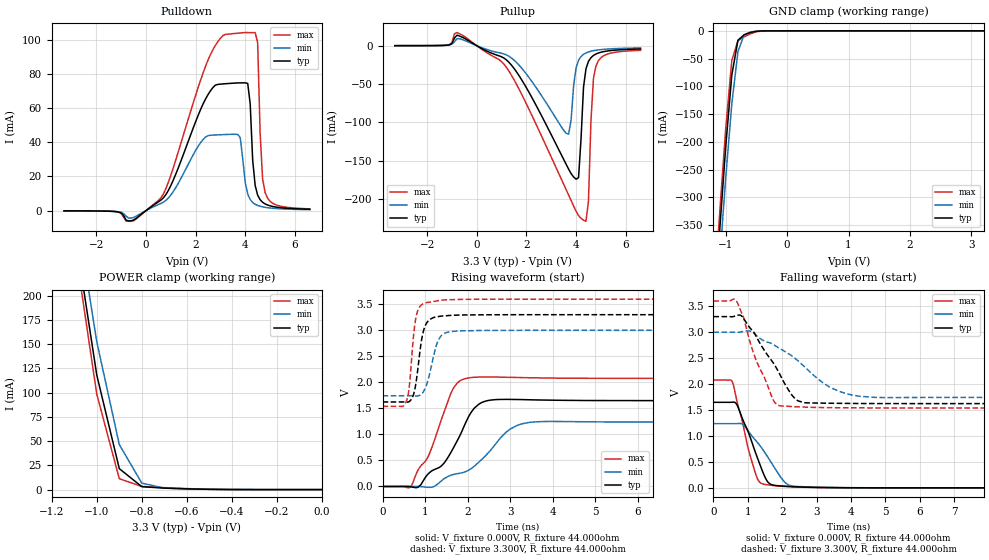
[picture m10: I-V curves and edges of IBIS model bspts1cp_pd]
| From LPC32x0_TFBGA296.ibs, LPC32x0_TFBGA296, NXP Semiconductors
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| |   Rev 0.20 IBIS Model Design Automation Generation   |
| |   N O N - S I L I C O N   C O R R E L A T E D   |
| |   This IBIS [Model] is pre-Beta tactical support   |
| |  Note: this IBIS [Model] contains clamp curves generated   |
| |   through simulation which should not be relied upon   |
| bspts1cp
|   Bidirectional Pad 3v3
|   3state Output
|   Plain Input
|   1ns Slew Rate control
|   CMOS
|   Programmable between
|   - (p1=0, p2=1) plain input
|   - (p1=0, p2=0) with Pull Up
|   - (p1=1, p2=1) with Pull Down
|   - (p1=1, p2=0) with Repeater
|   Characterized at Core 1.2V and I/O 3.3V
| Pull Down Mode (p1=1, p2=1)
[Model]   bspts1cp_pd | of bspts1cp
Model_type   I/O
Polarity   Non-Inverting
Enable   Active-Low
|  Reciever Thresholds
Vinl   = 0.36V
Vinh   = 0.84V
| AC Test Load Conditions
Vref   = 0
Cref   = 1.2e-11
Rref   = 1000000000
Vmeas   = 0.6
| [Process Range]   typical   min   max
| C_comp edge width   400.000ps   400.000ps   400.000ps
| C_comp Tstrobe   40.000fs   40.000fs   40.000fs
C_comp   2.380pF   2.240pF   2.550pF
[Temperature Range]   25   125   -40
[Voltage Range]   3.30V   3.00V   3.60V
[GND Clamp Reference]   0.00V   0.00V   0.00V
[Pulldown Reference]   0.00V   0.00V   0.00V
[POWER Clamp Reference]   3.30V   3.00V   3.60V
[Pullup Reference]   3.30V   3.00V   3.60V
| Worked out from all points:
|   slope of the pulldown table from 0 to 0.495 V, typ, clamps not added: 97.1 ohm
|   slope of the pullup table from 0 to 0.495 V, typ, clamps not added: 59.3 ohm
|   GND clamp passes 1 mA (typ) near -0.51 V on its own axis
|   POWER clamp passes 1 mA (typ) near -0.63 V on its own axis
|   rising waveform, V_fixture 0.000V, R_fixture 44.000ohm: 20-80 % time 779ps typ, 1.07ns min, 628ps max; typ from 0 V to 1.65 V
|   falling waveform, V_fixture 0.000V, R_fixture 44.000ohm: 20-80 % time 570ps typ, 781ps min, 474ps max; typ from 1.65 V to 0 V
|   rising waveform, V_fixture 3.300V, R_fixture 44.000ohm: 20-80 % time 175ps typ, 231ps min, 140ps max; typ from 1.62 V to 3.3 V
|   falling waveform, V_fixture 3.300V, R_fixture 44.000ohm: 20-80 % time 911ps typ, 1.48ns min, 670ps max; typ from 3.3 V to 1.62 V
[GND Clamp]
| ref voltage   0.00V   0.00V   0.00V
|   Voltage   I(typ)   I(min)   I(max)
-3.3V     -4.198A    -4.223A    -4.188A
-1.2V     -526mA     -577.5mA   -497.2mA
-1.1V     -363.6mA   -417.9mA   -332.6mA
-1V       -210.1mA   -266.3mA   -177.3mA
-900mV    -79.71mA   -131.5mA   -53.29mA
-800mV    -16.76mA   -37.38mA   -17.81mA
-700mV    -7.164mA   -7.263mA   -10.92mA
-600mV    -3.002mA   -2.202mA   -5.445mA
-500mV    -699uA     -571.9uA   -1.612mA
-400mV    -79uA      -96.04uA   -163.6uA
3.2V      50.82uA    25.42uA    83.99uA
[Power Clamp]   | Vtable = Vcc - Vpad
| ref voltage   3.30V   3.00V   3.60V
|   Voltage   I(typ)   I(min)   I(max)
-3.3V     4.52A      4.504A     4.537A
-1.1V     269.9mA    299.6mA    255.3mA
-1V       118.1mA    152.4mA    98.48mA
-900mV    21.62mA    46.52mA    11.25mA
-800mV    3.036mA    6.671mA    3.29mA
-700mV    1.546mA    1.556mA    2.017mA
-600mV    791.6uA    711.6uA    1.06mA
-400mV    91.28uA    94.64uA    124.4uA
0V        50.84uA    24.87uA    84.1uA
[Pulldown]
| ref voltage   0.00V   0.00V   0.00V
|   Voltage   I(typ)   I(min)   I(max)
-3.3V     -80.68uA   -69.9uA    -74.32uA
-600mV    -5.92mA    -4.329mA   -6.172mA
500mV     5.147mA    3.568mA    5.922mA
2.5V      67.8mA     43.83mA    87.99mA
3.7V      74.65mA    44.53mA    103.7mA
4V        74.69mA    16.44mA    104.1mA
4.2V      62.38mA    6.515mA    104mA
4.3V      29.48mA    4.769mA    104mA
4.5V      9.069mA    3.068mA    98.17mA
4.6V      6.413mA    2.587mA    45.15mA
4.8V      3.956mA    1.96mA     10.6mA
6.6V      844.8uA    597.5uA    1.056mA
[Pullup]   | Vtable = Vcc - Vpad
| ref voltage   3.30V   3.00V   3.60V
|   Voltage   I(typ)   I(min)   I(max)
-3.3V     39.4uA     37.84uA    38.83uA
-800mV    13.66mA    9.123mA    17.15mA
1V        -14.52mA   -9.936mA   -20.86mA
3.7V      -161.3mA   -115.5mA   -195.1mA
4V        -174.4mA   -29.02mA   -216.2mA
4.1V      -172.4mA   -19.17mA   -221.9mA
4.4V      -30.01mA   -9.422mA   -229.4mA
4.5V      -20.39mA   -8.135mA   -202.5mA
4.6V      -15.6mA    -7.195mA   -97.92mA
4.7V      -12.75mA   -6.48mA    -42.98mA
4.8V      -10.87mA   -5.92mA    -26.67mA
6.6V      -4.278mA   -2.929mA   -6.056mA
[Ramp]
R_load   = 44.000ohm
|   dV/dt(typ)   dV/dt(min)   dV/dt(max)
dV/dt_r   1.003V/795.000ps   754.478mV/1.100ns   1.260V/635.000ps
dV/dt_f   1.021V/900.000ps   769.240mV/1.445ns   1.253V/655.000ps
[Rising Waveform]  | cubic spline decimation from 2001 points
V_fixture   = 0.000V
R_fixture   = 44.000ohm
|   Time   V(typ)   V(min)   V(max)
0s        20.64nV    394.3nV    10.69nV
655ps     -4.509mV   428.1uV    -8.81mV
1.09ns    255.6mV    -17.26mV   603.8mV
1.445ns   447.6mV    146.5mV    1.426V
1.67ns    745mV      230.7mV    1.89V
1.965ns   1.242V     288.3mV    2.076V
2.37ns    1.625V     548.9mV    2.103V
2.915ns   1.673V     1.048V     2.097V
3.41ns    1.666V     1.225V     2.089V
10ns      1.648V     1.237V     2.076V
[Falling Waveform]  | cubic spline decimation from 2001 points
V_fixture   = 0.000V
R_fixture   = 44.000ohm
|   Time   V(typ)   V(min)   V(max)
0s        1.648V     1.237V     2.076V
555ps     1.65V      1.237V     2.038V
695ps     1.587V     1.238V     1.641V
1.075ns   967.6mV    1.04V      606.4mV
1.28ns    579.3mV    875mV      177mV
1.425ns   325.8mV    749.7mV    78.35mV
1.675ns   66.27mV    496.9mV    50.08mV
2.08ns    31.91mV    105.1mV    27.13mV
2.34ns    22mV       31.75mV    18.32mV
10ns      525.7nV    1.302uV    537.6nV
[Rising Waveform]  | cubic spline decimation from 2001 points
V_fixture   = 3.300V
V_fixture_min = 3.000V
V_fixture_max = 3.600V
R_fixture   = 44.000ohm
|   Time   V(typ)   V(min)   V(max)
0s        1.623V     1.742V     1.539V
555ps     1.622V     1.742V     1.629V
630ps     1.632V     1.742V     1.925V
730ps     1.769V     1.741V     2.902V
785ps     1.98V      1.739V     3.24V
920ps     2.821V     1.777V     3.49V
1.005ns   3.09V      1.889V     3.524V
1.31ns    3.263V     2.804V     3.57V
1.59ns    3.285V     2.972V     3.587V
10ns      3.299V     2.999V     3.598V
[Falling Waveform]  | cubic spline decimation from 2001 points
V_fixture   = 3.300V
V_fixture_min = 3.000V
V_fixture_max = 3.600V
R_fixture   = 44.000ohm
|   Time   V(typ)   V(min)   V(max)
0s        3.299V     2.999V     3.598V
670ps     3.321V     2.998V     3.602V
850ps     3.291V     3.011V     3.328V
1.25ns    2.912V     2.936V     2.448V
1.735ns   2.413V     2.766V     1.701V
1.885ns   2.247V     2.703V     1.59V
2.465ns   1.675V     2.445V     1.561V
3.385ns   1.63V      1.94V      1.545V
4.09ns    1.626V     1.781V     1.541V
10ns      1.623V     1.742V     1.539V
